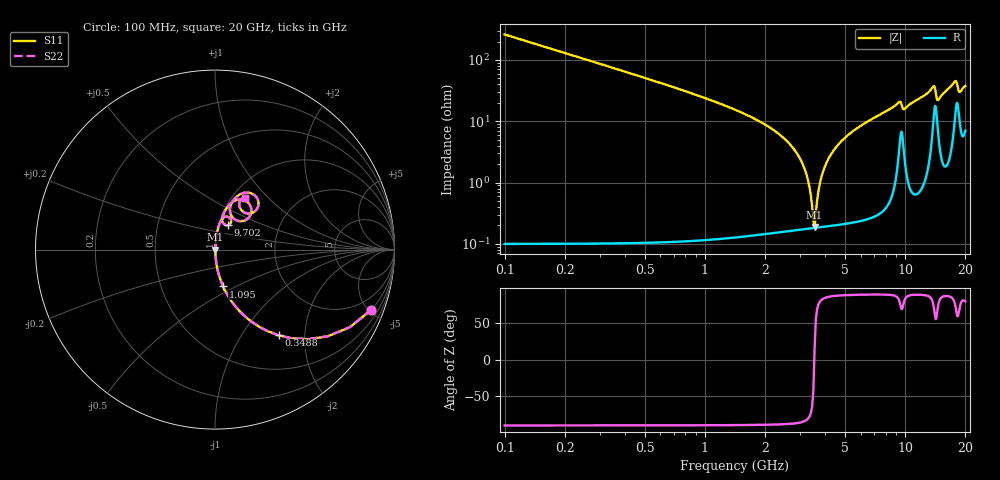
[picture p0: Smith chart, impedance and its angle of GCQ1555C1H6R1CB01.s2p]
!Murata Part Number: GCQ1555C1H6R1CB01
!These Parameters are Measured in Series Mode Connection
!Data Generated on Mar 13, 2026
!  o--ll--o
!Port1  Port2
!  o------o
!Operation Temp=25[degC], DC Bias Voltage=0[V]
!Freq. Start=100[MHz] Stop=20[GHz] 401[Steps]
# Hz S RI R 50
!Freq.(Hz) S11(Real) S11(Imag) S21(Real) S21(Imag) S12(Real) S12(Imag) S22(Real) S22(Imag)
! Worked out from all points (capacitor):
!   401 points, 100 MHz to 20 GHz, reference 50 ohm
!   read as one part in series: C = 6.1 pF near 199.5 MHz
!   lowest |Z| = 189 mohm at 3.533 GHz (marker M1)
!   series resonance near 3.521 GHz, so ESL is about 330 pH
!   S11 on the Smith chart (normalised r, x): 100 MHz: 1.00, -5.21; 348.8 MHz: 1.00, -1.48; 1.095 GHz: 1.00, -0.43; 9.702 GHz: 1.11, +0.31; 20 GHz: 1.14, +0.74
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1e8  0.8716 -0.3343  0.1284 0.3343  0.1284 0.3343  0.8716 -0.3343
3.4875e8  0.3545 -0.4777  0.6455 0.4777  0.6455 0.4777  0.3545 -0.4777
6.4725e8  0.1324 -0.3375  0.8676 0.3375  0.8676 0.3375  0.1324 -0.3375
1.095e9  0.0453 -0.2052  0.9547 0.2052  0.9547 0.2052  0.0453 -0.2052
2.83625e9  0.0027 -0.0322  0.9973 0.0322  0.9973 0.0322  0.0027 -0.0322
3.23425e9  0.00191 -0.0126  0.9981 0.0126  0.9981 0.0126  0.00191 -0.0126
3.43325e9  0.00181 -0.00372  0.9982 0.00372  0.9982 0.00372  0.00181 -0.00372
3.53275e9  0.00182 0.000509  0.9982 -0.000509  0.9982 -0.000509  0.00182 0.000509
3.881e9  0.0021 0.0145  0.9979 -0.0145  0.9979 -0.0145  0.0021 0.0145
4.3785e9  0.00305 0.0326  0.9969 -0.0326  0.9969 -0.0326  0.00305 0.0326
5.274e9  0.00602 0.0618  0.994 -0.0618  0.994 -0.0618  0.00602 0.0618
6.7665e9  0.0139 0.1053  0.9861 -0.1053  0.9861 -0.1053  0.0139 0.1053
9.30375e9  0.0651 0.1835  0.9349 -0.1835  0.9349 -0.1835  0.0651 0.1835
9.70175e9  0.0731 0.1368  0.9269 -0.1368  0.9269 -0.1368  0.0731 0.1368
1.005e10  0.0423 0.1541  0.9577 -0.1541  0.9577 -0.1541  0.0423 0.1541
1.338325e10  0.1154 0.2748  0.8846 -0.2748  0.8846 -0.2748  0.1154 0.2748
1.39305e10  0.1923 0.2524  0.8077 -0.2524  0.8077 -0.2524  0.1923 0.2524
1.45275e10  0.1065 0.1708  0.8935 -0.1708  0.8935 -0.1708  0.1065 0.1708
1.67165e10  0.1303 0.3024  0.8697 -0.3024  0.8697 -0.3024  0.1303 0.3024
1.7811e10  0.2274 0.2963  0.7726 -0.2963  0.7726 -0.2963  0.2274 0.2963
1.865675e10  0.1526 0.2139  0.8474 -0.2139  0.8474 -0.2139  0.1526 0.2139
2e10  0.166 0.2889  0.834 -0.2889  0.834 -0.2889  0.166 0.2889
